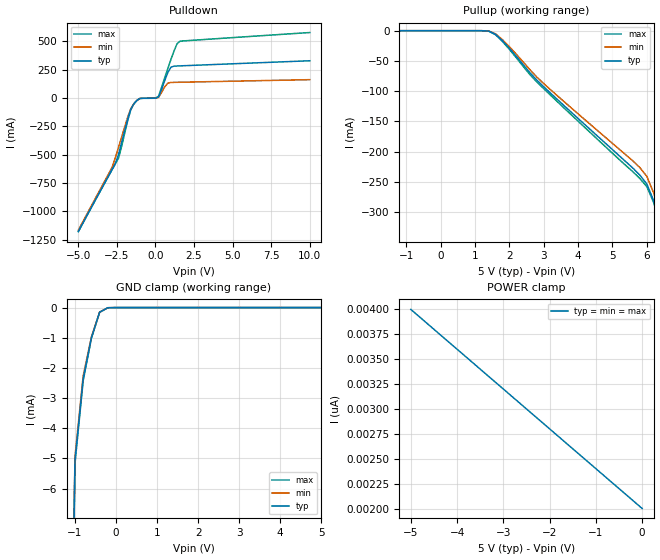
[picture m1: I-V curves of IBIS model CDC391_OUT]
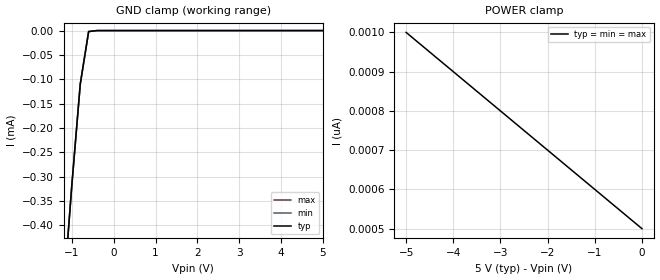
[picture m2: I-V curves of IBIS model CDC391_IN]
|   TEXAS INSTRUMENTS INCORPORATED
|   BuS Solutions Group
|   IBIS Model of CDC391
|   5.0-V 1-LINE to 6-LINE Clock DRIVER
|   16-pin (D or DB) Package
[IBIS Ver]   2.1
[File Name]   cdc391.ibs
[File Rev]   1.0
[Date]   09/08/00
[Source]   File originated at Texas Instruments, Inc.
[Notes]   The following is an IBIS list for the CDC329.
|   - All test data contained in this file are derived from
|   hspice(tm) simulations.
|   - File created by Dung Nguyen, BuS Solutions Applications.
[Disclaimer] Property of Texas Instruments Incorporated.  Unauthorized
   reproduction and/or distribution is strictly prohibited.
   This product is protected under copyright law.
   Created 2000, (C) Copyright 2000, Texas Instruments Inc.,
   All Rights Reserved
   UNLESS THERE IS A SIGNED, WRITTEN AGREEMENT TO THE
   CONTRARY, TEXAS INSTRUMENTS ("TI") IS PROVIDING THE IBIS
   MODELS "AS IS" AND WITHOUT ANY WARRANTY, EXPRESSED OR
   IMPLIED.  TI assumes no liability for:
   1) the accuracy of the IBIS models provided to your
   company;
   2) the proper functioning of these IBIS models in your
   design or for any resulting applications; or
   3) infringement of patents, copyrights or intellectual
   property rights resulting from your use of these IBIS
   models.
   TI provides IBIS Models as a service to our customers.
   You and your company shall not distribute, sell or give
   these models to anyone else without prior written
   permission from TI.
   TI reserves the right to make changes to our products or
   to discontinue any semiconductor product or service
   without notice, and advises our customers to obtain the
   latest version of relevant information to verify, before
   placing orders, that the information being relied on is
   current.
   Please be aware that your receipt and use of the IBIS
   information provided shall serve as acceptance of these
   terms and conditions.  If you do not accept these terms,
   you should return or destroy the IBIS models and any
   other accompanying information immediately.
[Component]   CDC391(5.0V_CLOCK_DRIVER)
[Manufacturer]  Texas Instruments, Inc.
[Package]
|   typ   min   max
R_pkg   0.041631   0.03463   0.0485908
L_pkg   3.1471nH   2.16389nH   4.21505nH
C_pkg   0.197875pF   0.0884942pF   0.391802pF
[Pin]   signal_name   model_name
1   GND   GND
2   1Y2   CDC391_OUT
3   1Y3   CDC391_OUT
4   GND   GND
5   2Y1   CDC391_OUT
6   2Y2   CDC391_OUT
7   GND   CDC391_OUT
8   3Y1   CDC391_OUT
9   OE   CDC391_IN
10   3T/C   CDC391_OUT
11   VCC   POWER
12   A   CDC391_IN
13   2T/C   CDC391_IN
14   VCC   POWER
15   1T/C   CDC391_IN
16   1Y1   CDC391_OUT
| Models and submodels in the file (2): CDC391_OUT (3-state), CDC391_IN (Input)
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|   Model CDCVF2505_OUT
[Model]   CDC391_OUT
Model_type   3-state
Polarity   Non-Inverting
Enable   Active-High
Vmeas = 2.5V   |Vref for timing measurements.
Cref = 50pF   |load capacitance for timing spec.
Rref = 500   |500 Ohm to GND.
Vref = 0   |Timing specification test load voltage; GND
|   typ   min   max
C_comp   4.8pF   NA   NA
[Voltage range]   5.0   4.75   5.25
[Temperature range]   25   -40   85
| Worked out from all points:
|   slope of the pulldown table from 0 to 0.75 V, typ, clamps not added: 3.6 ohm
|   GND clamp passes 1 mA (typ) near -0.60 V on its own axis
| Notes: (1) Vtable = Vcc - Voutput
|   (2) Pullup data includes the effects of the ESD
|   clamping circuitry
[Pullup]
|   Voltage  I(typ)   I(min)   I(max)
-5V       3.5nA      3.5nA      3.5nA
1.4V      -625.2uA   -474.6uA   -781uA
1.6V      -6.009mA   -5.115mA   -6.766mA
1.8V      -16.48mA   -14.77mA   -17.76mA
2.6V      -69.63mA   -64.58mA   -72.65mA
3V        -92.71mA   -87.42mA   -95.82mA
5.8V      -239.1mA   -226.7mA   -244.6mA
6V        -253.8mA   -241.1mA   -258mA
6.2V      -281.5mA   -268.7mA   -284.5mA
6.4V      -319.7mA   -306.8mA   -322.4mA
6.6V      -361.7mA   -348.6mA   -364.6mA
10V       -1.183A    -1.175A    -1.186A
[Pulldown]
| Volt   I(typ)   I(min)   I(max)
-5V       -1.178A    -1.166A    -1.179A
-2.8V     -627mA     -608mA     -630.2mA
-2.4V     -500.8mA   -437.8mA   -532.5mA
-1.8V     -186.2mA   -169.5mA   -200.6mA
-1.6V     -100.4mA   -95.44mA   -105mA
-1.4V     -51.97mA   -51.39mA   -52.64mA
-1V       -4.764mA   -4.427mA   -5.305mA
200mV     8.622mA    4.39mA     15.27mA
600mV     152.3mA    97.3mA     177.4mA
1V        270mA      136mA      337.5mA
1.4V      281mA      137.3mA    477.3mA
10V       327.1mA    160.5mA    575.9mA
[GND Clamp]
|   Voltage   I(typ)   I(min)   I(max)
-5V       -1.18A     -1.17A     -1.18A
-1.2V     -22.2mA    -22.1mA    -22.3mA
-1V       -5.06mA    -4.94mA    -5.17mA
-800mV    -2.35mA    -2.26mA    -2.42mA
-600mV    -998uA     -974uA     -1.02mA
-400mV    -154uA     -153uA     -155uA
-200mV    -5.71uA    -5.71uA    -5.71uA
5V        170nA      170nA      170nA
[POWER Clamp]
|   Voltage   I(typ)   I(min)   I(max)
-5V       4nA        4nA        4nA
-4.8V     3.92nA     3.92nA     3.92nA
-4.2V     3.68nA     3.68nA     3.68nA
0V        2nA        2nA        2nA
[ramp]
| variable   typ   min   max
dV/dt_r   1.6E+00/4.1E-10   1.554E00/4.10E-10   1.657E+00/4.36E-10
dV/dt_f   2.77E+00/3.4E-10   2.748E00/3.67E-10   2.791E+00/3.43E-10
|   Model CDCVF2505_IN
[Model]   CDC391_IN
Model_type   Input
Polarity   Non-Inverting
Vinl = 0.8V
Vinh = 2.0V
|   typ   min   max
C_comp   2.8pF   NA   NA
[Voltage Range]   5.0   4.75   5.25
[Temperature range]   25   -40   85
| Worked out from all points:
|   GND clamp passes 1 mA (typ) near -1.58 V on its own axis
[GND Clamp]
|   Voltage   I(typ)   I(min)   I(max)
-5V       -5.64mA    -5.64mA    -5.64mA
-1.2V     -542uA     -541uA     -542uA
-1V       -316uA     -316uA     -316uA
-800mV    -110uA     -110uA     -110uA
-600mV    -2uA       -2uA       -2.01uA
-400mV    -1.42nA    -1.42nA    -1.43nA
5V        500pA      500pA      500pA
[POWER Clamp]
|  Voltage   I(typ)   I(min)   I(max)
-5V       1nA        1nA        1nA
-4.8V     980pA      980pA      980pA
-4.2V     920pA      920pA      920pA
0V        500pA      500pA      500pA
